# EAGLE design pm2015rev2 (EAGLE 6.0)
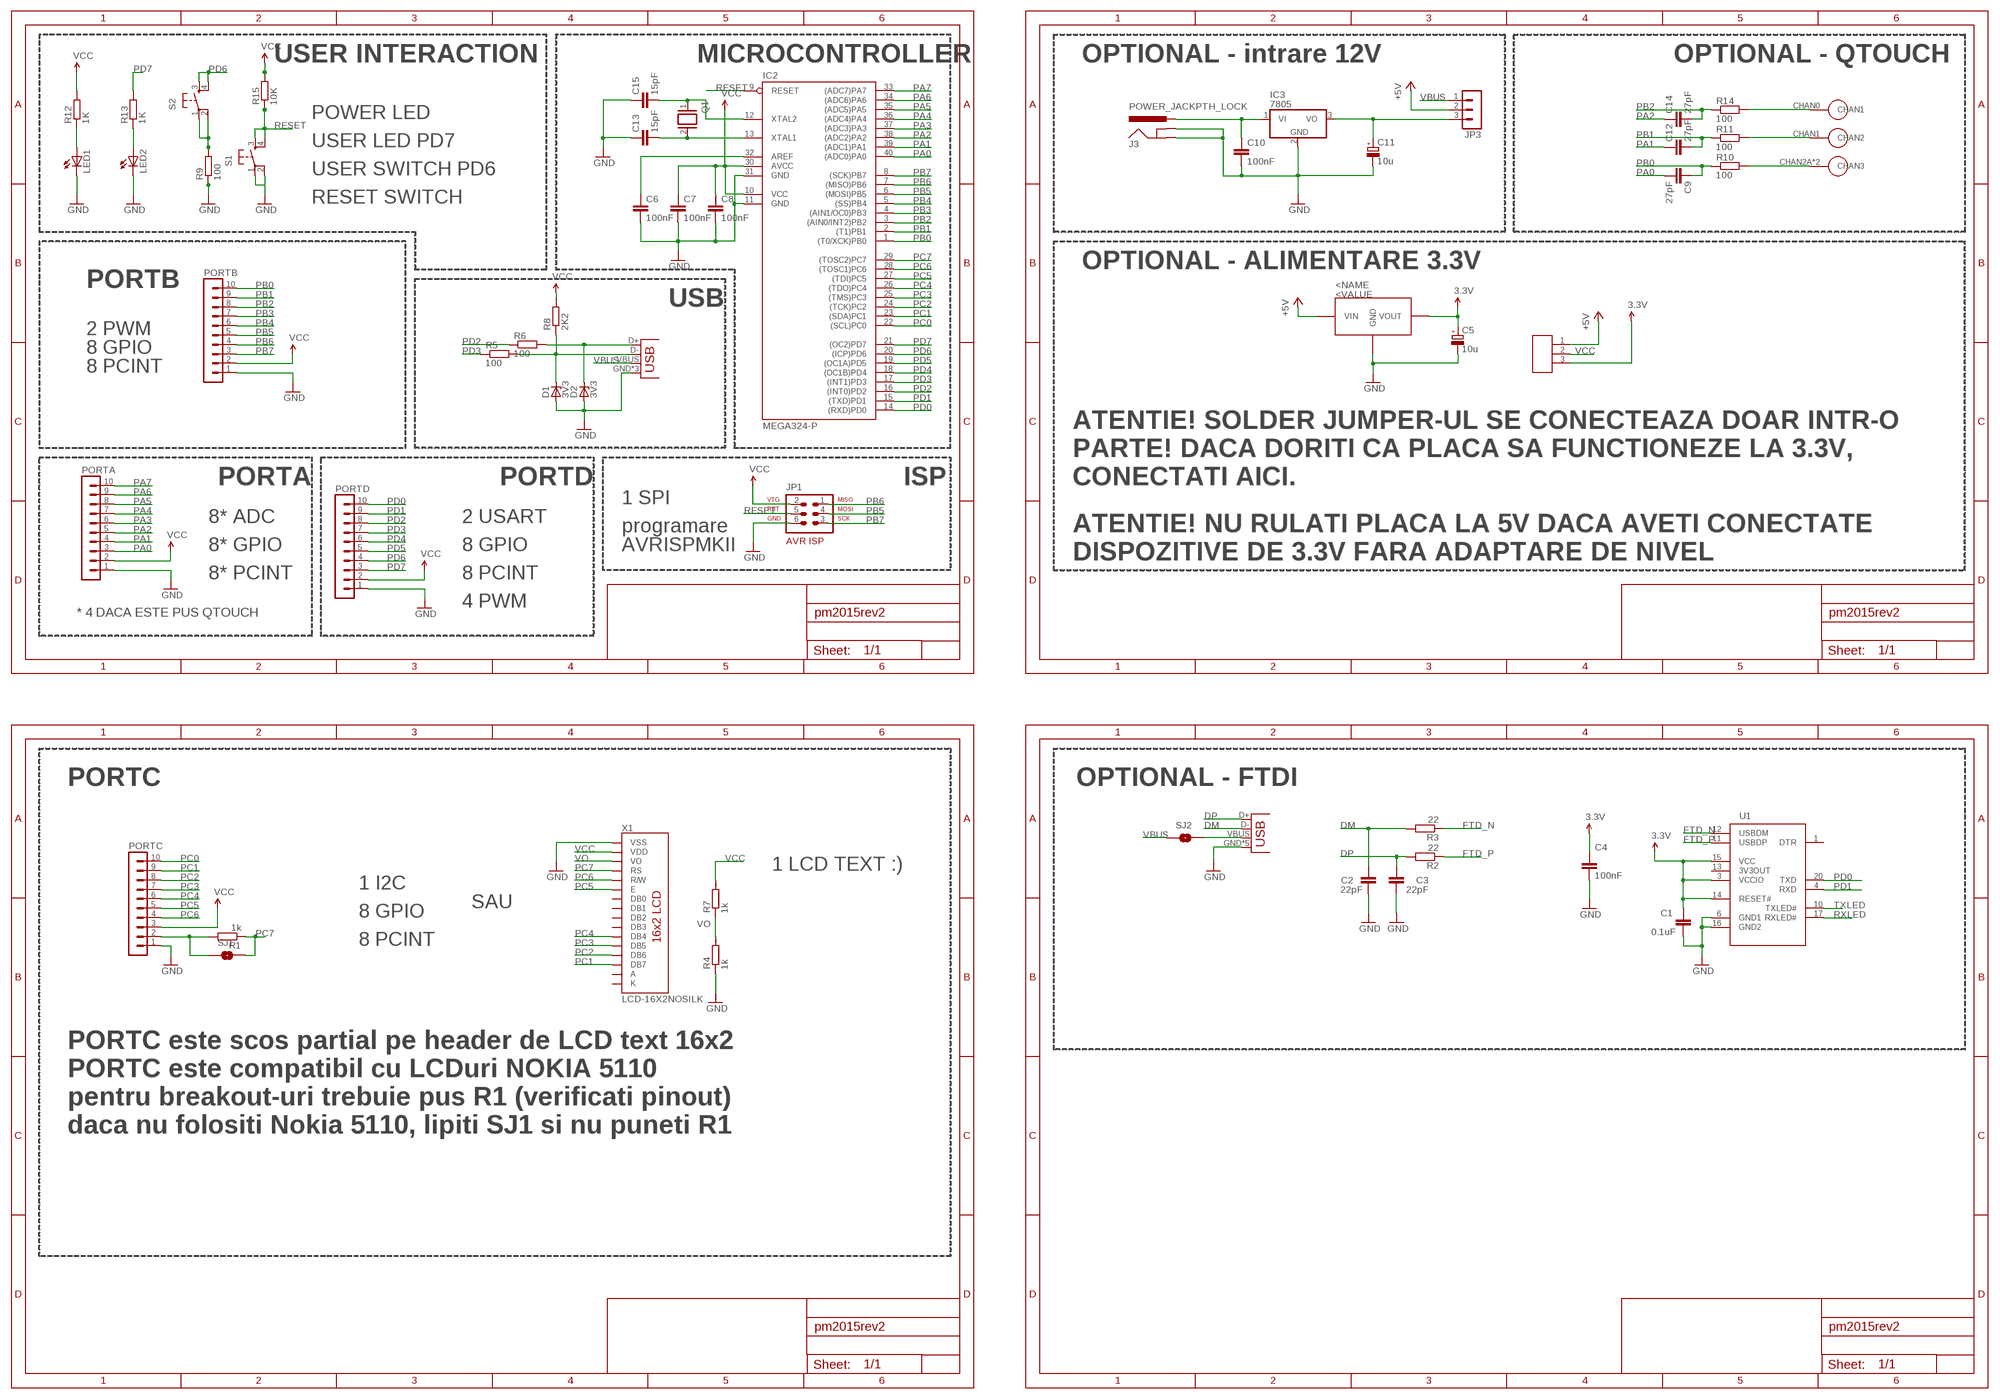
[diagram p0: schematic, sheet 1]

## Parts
C1  0.1uF  C-EUC0603  [C0603]
C2  22pF  C-EUC0603  [C0603]
C3  22pF  C-EUC0603  [C0603]
C4  100nF  C-EUC0603  [C0603]
C5  10u  CPOL-EUE2.5-5  [E2,5-5]
C6  100nF  C-EUC_PM  [C025-025X050]
C7  100nF  C-EUC_PM  [C025-025X050]
C8  100nF  C-EUC_PM  [C025-025X050]
C9  27pF  C-EUC1206  [C1206]
C10  100nF  C-EU025-025X050  [C025-025X050@1]
C11  10u  CPOL-EUE2.5-5  [E2,5-5]
C12  27pF  C-EUC1206  [C1206]
C13  15pF  C-EUC_PM  [C025-025X050]
C14  27pF  C-EUC1206  [C1206]
C15  15pF  C-EUC_PM  [C025-025X050]
D1  3V3  ZENER-DIODEDO34-7  [DO34Z7]
D2  3V3  ZENER-DIODEDO34-7  [DO34Z7]
IC1  LE33  [TO92]
IC2  MEGA324-P  MEGA16-P  [DIL40]
IC3  7805  7805TNH  [TO22H_NOHOLE]
J1  USBMICROUSB  [ZX62D-B-5PA8]
J2  USBPTH  [USB-B-PTH]
J3  POWER_JACKPTH_LOCK  [POWER_JACK_PTH_LOCK]
JP1  AVR-ISP-6  [AVR-ISP-6]
JP2  SJUMPER  [SJUMPER_PACK]
JP3  MA03-1  [MA03-1]
LED1  TLLR4400  [LED3MM]
LED2  TLLR4400  [LED3MM]
PORTA  MA10-1  [MA10-1]
PORTB  MA10-1  [MA10-1]
PORTC  MA10-1  [MA10-1]
PORTD  MA10-1  [MA10-1]
Q1  XTAL/S  [QS]
R1  1k  R-EU_0204/7  [0204/7]
R2  22  R-EU_R0603  [R0603]
R3  22  R-EU_R0603  [R0603]
R4  1k  R-EU_0204/7  [0204/7]
R5  100  R-EU_0204/7  [0204/7]
R6  100  R-EU_0204/7  [0204/7]
R7  1k  R-EU_0204/7  [0204/7]
R8  2K2  R-EU_0204/7  [0204/7]
R9  100  R-EU_0204/7  [0204/7]
R10  100  R-EU_M1206  [M1206]
R11  100  R-EU_M1206  [M1206]
R12  1K  R-EU_0204/7  [0204/7]
R13  1K  R-EU_0204/7  [0204/7]
R14  100  R-EU_M1206  [M1206]
R15  10K  R-EU_0204/7  [0204/7]
S1  TAC_SWITCHPTH  [TACTILE-PTH]
S2  TAC_SWITCHPTH  [TACTILE-PTH]
SJ1  SOLDERJUMPERNC  [SJ-NC]
SJ2  SOLDERJUMPERNC  [SJ-NC]
U1  FT231XS  [SSOP20]
U$1  QT_SLIDER  [QT_SLIDER]
X1  LCD-16X2NOSILK  [LCD-16X2_NOSILK]

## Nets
3.3V: C1.1 C4.1 C5.+ IC1.3(VOUT) JP2.3 U1.3(VCCIO) U1.14(RESET#) U1.15(VCC)
+5V: IC1.1(VIN) JP2.1 JP3.2
DM: C2.2 J1.D- R3.2
DP: C3.2 J1.D+ R2.2
FTD_N: R3.1 U1.12(USBDM)
FTD_P: R2.1 U1.11(USBDP)
GND: C1.2 C2.1 C3.1 C4.2 C5.- C6.2 C7.2 C8.2 C10.2 C11.- C13.1 C15.1 D1.A D2.A IC1.2(GND) IC2.11(GND) IC2.31(GND) IC3.2(GND) J1.GND J1.P$8(GND) J1.P$9(GND) J1.P$10(GND) J1.P$11(GND) J2.GND J2.P$1(GND) J2.P$2(GND) J3.GND J3.GNDBREAK JP1.6 LED1.K(C) LED2.K(C) PORTA.1 PORTB.1 PORTC.1 PORTD.1 R4.1 R9.1 S1.1 S1.2 U1.6(GND1) U1.16(GND2) X1.1(VSS)
N$1: LED2.A R13.1
N$2: LED1.A R12.1
N$3: PORTC.2 R1.2 SJ1.1
N$4: J1.VBUS SJ2.2
N$5: R14.2 U$1.CHAN0(CHAN1)
N$6: R11.2 U$1.CHAN1(CHAN2)
N$7: R10.2 U$1.CHAN2A(CHAN3) U$1.CHAN2B(CHAN3)
N$14: D2.C J2.D+ R6.2
N$15: D1.C J2.D- R5.2 R8.1
N$16: C10.1 IC3.1(VI) J3.PWR
N$17: R9.2 S2.1 S2.2
N$18: C11.+ IC3.3(VO) JP3.3
N$20: C6.1 IC2.32(AREF)
N$21: C13.2 IC2.13(XTAL1) Q1.2
N$22: C15.2 IC2.12(XTAL2) Q1.1
PA0: C9.2 IC2.40((ADC0)PA0) PORTA.3
PA1: C12.1 IC2.39((ADC1)PA1) PORTA.4
PA2: C14.1 IC2.38((ADC2)PA2) PORTA.5
PA3: IC2.37((ADC3)PA3) PORTA.6
PA4: IC2.36((ADC4)PA4) PORTA.7
PA5: IC2.35((ADC5)PA5) PORTA.8
PA6: IC2.34((ADC6)PA6) PORTA.9
PA7: IC2.33((ADC7)PA7) PORTA.10
PB0: C9.1 IC2.1((T0/XCK)PB0) PORTB.10 R10.1
PB1: C12.2 IC2.2((T1)PB1) PORTB.9 R11.1
PB2: C14.2 IC2.3((AIN0/INT2)PB2) PORTB.8 R14.1
PB3: IC2.4((AIN1/OC0)PB3) PORTB.7
PB4: IC2.5((SS)PB4) PORTB.6
PB5: IC2.6((MOSI)PB5) JP1.4 PORTB.5
PB6: IC2.7((MISO)PB6) JP1.1 PORTB.4
PB7: IC2.8((SCK)PB7) JP1.3 PORTB.3
PC0: IC2.22((SCL)PC0) PORTC.10
PC1: IC2.23((SDA)PC1) PORTC.9 X1.14(DB7)
PC2: IC2.24((TCK)PC2) PORTC.8 X1.13(DB6)
PC3: IC2.25((TMS)PC3) PORTC.7 X1.12(DB5)
PC4: IC2.26((TDO)PC4) PORTC.6 X1.11(DB4)
PC5: IC2.27((TDI)PC5) PORTC.5 X1.6(E)
PC6: IC2.28((TOSC1)PC6) PORTC.4 X1.5(R/W)
PC7: IC2.29((TOSC2)PC7) R1.1 SJ1.2 X1.4(RS)
PD0: IC2.14((RXD)PD0) PORTD.10 U1.20(TXD)
PD1: IC2.15((TXD)PD1) PORTD.9 U1.4(RXD)
PD2: IC2.16((INT0)PD2) PORTD.8 R6.1
PD3: IC2.17((INT1)PD3) PORTD.7 R5.1
PD4: IC2.18((OC1B)PD4) PORTD.6
PD5: IC2.19((OC1A)PD5) PORTD.5
PD6: IC2.20((ICP)PD6) PORTD.4 S2.3 S2.4
PD7: IC2.21((OC2)PD7) PORTD.3 R13.2
RESET: IC2.9(RESET) JP1.5 R15.1 S1.3 S1.4
RXLED: U1.17(RXLED#)
TXLED: U1.10(TXLED#)
VBUS: J2.VBUS JP3.1 SJ2.1
VCC: C7.1 C8.1 IC2.10(VCC) IC2.30(AVCC) JP1.2 JP2.2 PORTA.2 PORTB.2 PORTC.3 PORTD.2 R7.2 R8.2 R12.2 R15.2 X1.2(VDD)
VO: R4.2 R7.1 X1.3(VO)
Unconnected: U1.1(DTR) U1.13(3V3OUT) X1.7(DB0) X1.8(DB1) X1.9(DB2) X1.10(DB3)

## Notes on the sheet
- USER INTERACTION | MICROCONTROLLER | OPTIONAL - intrare 12V | OPTIONAL - QTOUCH
- POWER LED
- USER LED PD7
- USER SWITCH PD6
- RESET SWITCH
- OPTIONAL - ALIMENTARE 3.3V
- PORTB
- USB
- 2 PWM
- 8 GPIO
- 8 PCINT
- ATENTIE! SOLDER JUMPER-UL SE CONECTEAZA DOAR INTR-O
- PARTE! DACA DORITI CA PLACA SA FUNCTIONEZE LA 3.3V,
- PORTA | PORTD | ISP | CONECTATI AICI.
- 1 SPI
- 8* ADC | 2 USART
- programare | ATENTIE! NU RULATI PLACA LA 5V DACA AVETI CONECTATE
- 8* GPIO | 8 GPIO | AVRISPMKII
- DISPOZITIVE DE 3.3V FARA ADAPTARE DE NIVEL
- 8* PCINT | 8 PCINT
- 4 PWM
- * 4 DACA ESTE PUS QTOUCH
- PORTC | OPTIONAL - FTDI
- 1 LCD TEXT :)
- 1 I2C
- SAU
- 8 GPIO
- 8 PCINT
- PORTC este scos partial pe header de LCD text 16x2
- PORTC este compatibil cu LCDuri NOKIA 5110
- pentru breakout-uri trebuie pus R1 (verificati pinout)
- daca nu folositi Nokia 5110, lipiti SJ1 si nu puneti R1

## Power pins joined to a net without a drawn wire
A: X1.15(A)
K: X1.16(K)

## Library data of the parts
C1-C4 C9 C10 C12 C14 = resistor:C-EU: CAPACITOR, European symbol
C5 C11 = resistor:CPOL-EU: POLARIZED CAPACITOR, European symbol
C6-C8 C13 C15 = 0andrei_custom:C-EU: CAPACITOR, European symbol
D1 D2 = diode:ZENER-DIODE: Z-Diode
IC1 = 0andrei_custom:LE33
IC2 = atmel:MEGA16-P: MICROCONTROLLER 16 Kbytes FLASH 1 kbytes SRAM 512 bytes EEPROM USART 8-channel 10 bit ADC Source: avr.lbr; MPN: ATMEGA16-16PU; OC_FARNELL: 9171142; OC_NEWARK: 01M6885
IC3 = 0andrei_custom:78*: Positive VOLTAGE REGULATOR Source: http://cache.national.com/ds/LM/LM78L05.pdf http://www.fairchildsemi.com/ds/LM/LM7805.pdf
J1 J2 = 0andrei_custom:USB: USB Connectors USB-B-PTH is fully proven SKU : PRT-00139 USB-miniB is fully proven SKU : PRT-00587 USB-A-PCB is untested. USB-A-H is throughly reviewed, but untested. Spark Fun Electronics SKU : PRT-00437 USB-B-SMT is throughly reviewed, but untested. Needs silkscreen touching up. USB-A-S has not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
J3 = SparkFun-Connectors:POWER_JACK: Power Jack This is the standard 5.5mm barrel jack for power. The PTH is the most common, proven, reliable, footprint. The Slot footprint only works if the mill layer is transmitted to the PCB fab house so be warned. Spark Fun Electronics SKU : PRT-00119 SMT: CONN-08106 Mating wall wart : TOL-00298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
JP1 = 0andrei_custom:AVR-ISP-6: AVR ISP-6 Serial Programming Header
JP2 = 0andrei_custom:SJUMPER
JP3 = con-lstb:MA03-1: PIN HEADER; OC_FARNELL: unknown; OC_NEWARK: unknown
LED1 LED2 = led:TLLR4400: Low Current (2mA) LED 3 mm Tinted Diffused Package color RED; MF: VISHAY SEMICONDUCTOR; OC_FARNELL: 1612437
PORTA PORTB PORTC PORTD = con-lstb:MA10-1: PIN HEADER; OC_FARNELL: unknown; OC_NEWARK: unknown
Q1 = special:XTAL/S: CRYSTAL
R1 R4-R9 R12 R13 R15 = 0andrei_custom:R-EU_: RESISTOR, European symbol
R2 R3 R10 R11 R14 = resistor:R-EU_: RESISTOR, European symbol
S1 S2 = SparkFun:TAC_SWITCH: Momentary Switch Button commonly used for reset or general input. Spark Fun Electronics SKU : COM-00097
SJ1 SJ2 = SparkFun-3-2-07:SOLDERJUMPER: Solder Jumper
U1 = 0andrei_custom:FT231XS
U$1 = 0andrei_custom:QT_SLIDER
X1 = 0andrei_custom:LCD-16X2: Standard text-only 16x2 parallel input LCD

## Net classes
1 power: width 0.61 mm

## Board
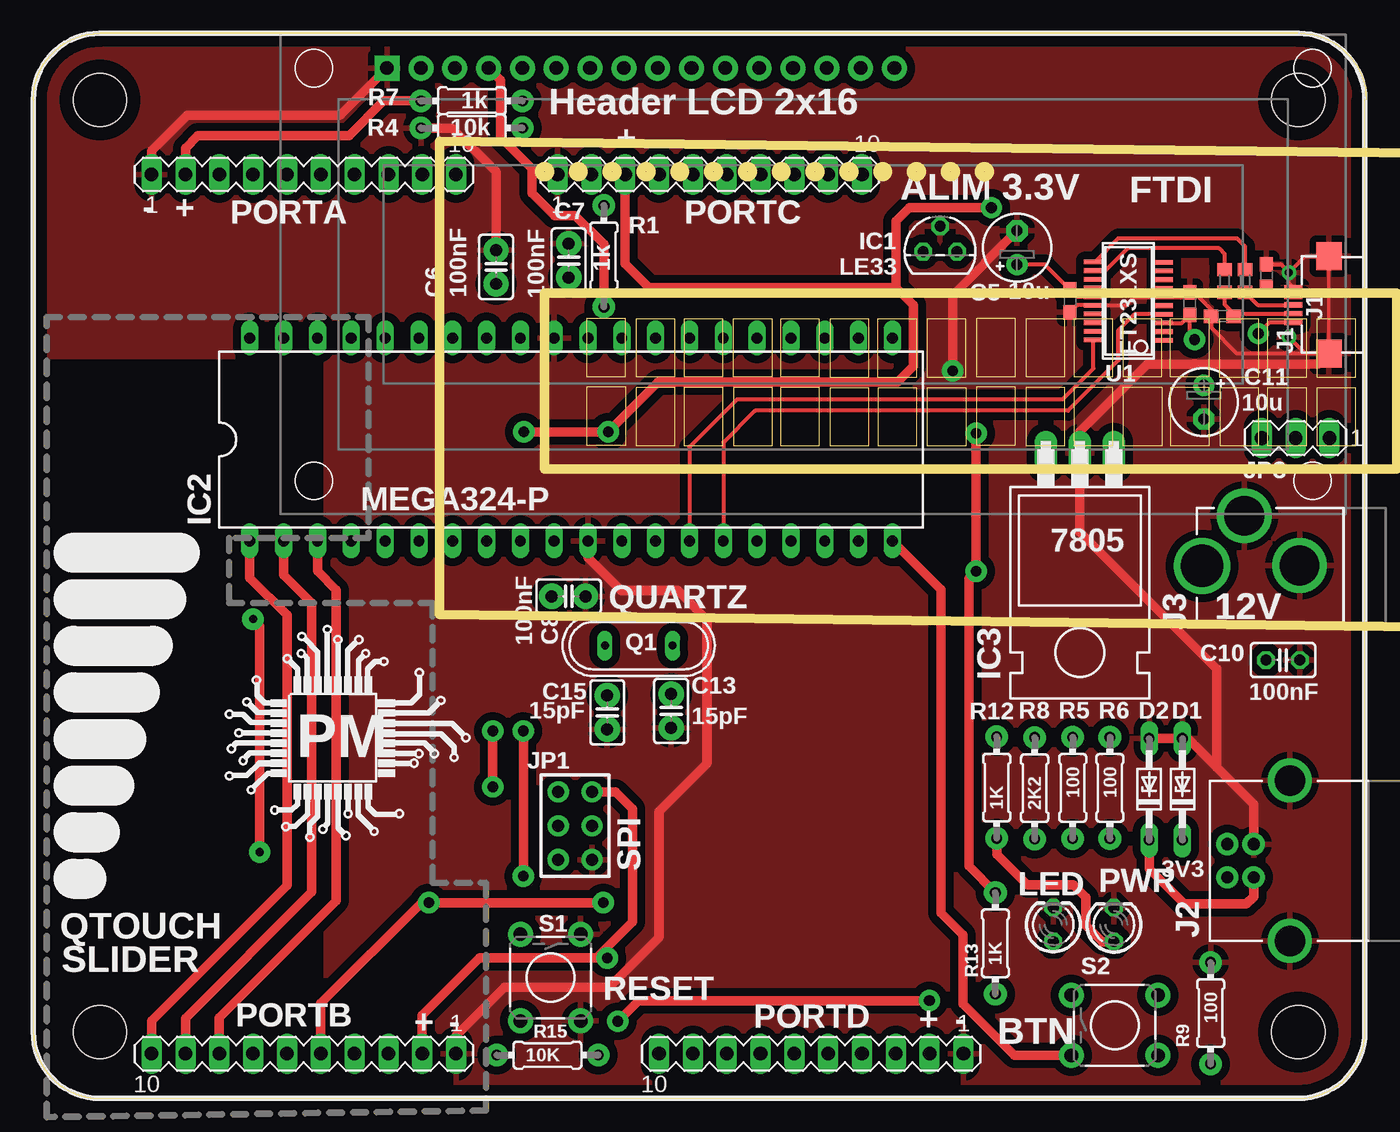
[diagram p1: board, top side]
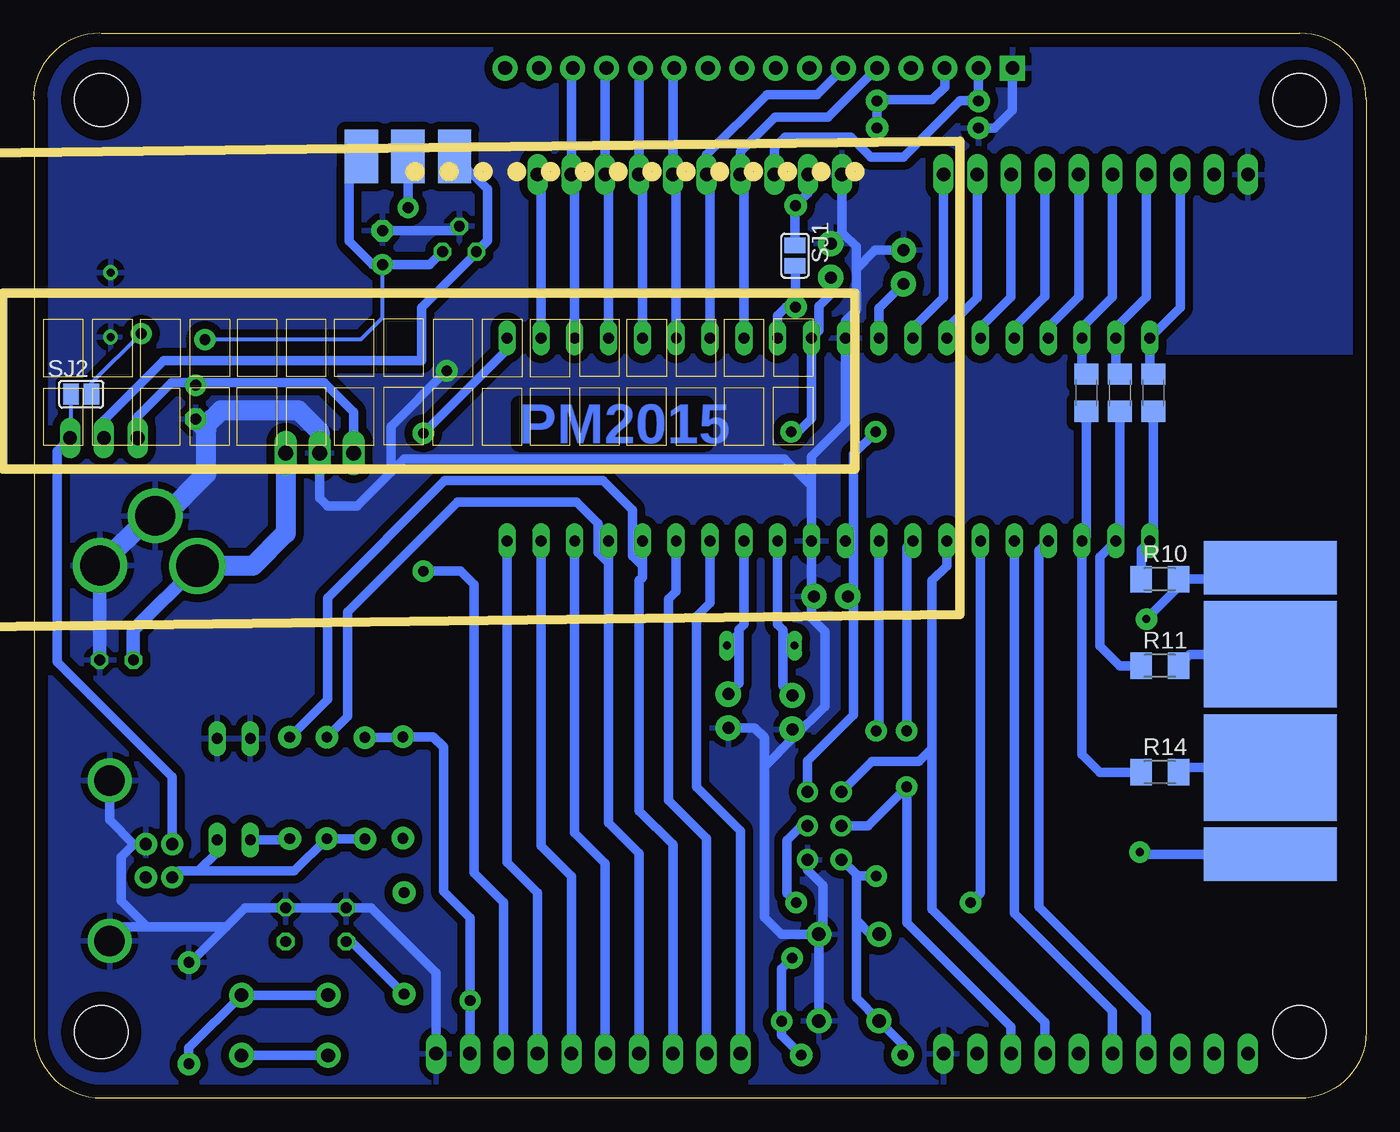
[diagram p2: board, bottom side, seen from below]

Size 100.1 x 80 mm. Coordinates in mm from the lower left corner, seen from the top.
Outline: 100,75 100,5 arc-90 95,0 5,0 arc-90 0,5 0,75 arc-90 5,80 95,80
Outline: 95.1,80 arc-90 100.1,75
Copper layers (1*16): Top 0.035mm / dielectric 1.5mm / Bottom 0.035mm
Design rules: minimum track width 10mil, minimum drill 0.6mm, track to track 0.25mm, track to pad 10mil, pad to pad 0.2mm, via to via 10mil, smd to smd 0mil, copper to edge 40mil, drill to drill 10mil, minimum pad ring 10mil, minimum via ring 8mil, stop-mask expansion 0mil, vias tented up to drill 0mil, thermal gap 20mil
Holes 4 mm at 95,75 5,5 5,75 95,5
Milling: area 38,69.3 to 38.8,70; area 40.6,69.3 to 41.3,70; area 43.1,69.3 to 43.8,70; area 45.7,69.3 to 46.4,70; area 48.2,69.3 to 48.9,70; area 50.7,69.3 to 51.5,70; area 53.3,69.3 to 54,70; area 55.8,69.3 to 56.5,70; area 58.4,69.3 to 59.1,70; area 60.9,69.3 to 61.6,70; area 63.4,69.3 to 64.2,70; area 66,69.3 to 66.7,70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; 8 lines

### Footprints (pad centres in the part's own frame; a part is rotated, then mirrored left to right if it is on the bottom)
C0603 = smd 1.1 x 1: 1 -0.85,0; 2 0.85,0
E2,5-5 = drill 0.813 pad 1.6: + -1.27,0 | drill 0.813 pad 1.6 octagon: - 1.27,0
C025-025X050 = drill 0.9 pad 1.9: 1 -1.27,0; 2 1.27,0
C1206 = smd 1.6 x 1.8: 1 -1.4,0; 2 1.4,0
C025-025X050@1 = drill 0.813 octagon: 1 -1.27,0; 2 1.27,0
DO34Z7 = drill 0.813 long: A 3.81,0; C -3.81,0
TO92 = drill 0.813 octagon: 1 -1.27,0; 2 0,1.905; 3 1.27,0
DIL40 = drill 0.813 long: 1 -24.13,-7.62; 2 -21.59,-7.62; 3 -19.05,-7.62; 4 -16.51,-7.62; 5 -13.97,-7.62; 6 -11.43,-7.62; 7 -8.89,-7.62; 8 -6.35,-7.62; 9 -3.81,-7.62; 10 -1.27,-7.62; 11 1.27,-7.62; 12 3.81,-7.62; 13 6.35,-7.62; 14 8.89,-7.62; 15 11.43,-7.62; 16 13.97,-7.62; 17 16.51,-7.62; 18 19.05,-7.62; 19 21.59,-7.62; 20 24.13,-7.62; 21 24.13,7.62; 22 21.59,7.62; 23 19.05,7.62; 24 16.51,7.62; 25 13.97,7.62; 26 11.43,7.62; 27 8.89,7.62; 28 6.35,7.62; 29 3.81,7.62; 30 1.27,7.62; 31 -1.27,7.62; 32 -3.81,7.62; 33 -6.35,7.62; 34 -8.89,7.62; 35 -11.43,7.62; 36 -13.97,7.62; 37 -16.51,7.62; 38 -19.05,7.62; 39 -21.59,7.62; 40 -24.13,7.62
TO22H_NOHOLE = drill 1.118 long: 1 -2.54,-10.16; 2 0,-10.16; 3 2.54,-10.16
ZX62D-B-5PA8 = smd 0.4 x 1.35: D+ 0,2.675; D- -0.65,2.675; GND 1.3,2.675; ID 0.65,2.675; VBUS -1.3,2.675 | drill 0.6: P$8 -2.425,3; P$9 2.425,3 | smd 2.1 x 1.9: P$10 -3.65,0; P$11 3.65,0
USB-B-PTH = drill 0.914 pad 1.676: D+ 0,1.25; D- 1.981,1.25; GND 0,-1.25; VBUS 1.981,-1.25 | drill 2.286: P$1 -2.718,-6.02; P$2 -2.718,6.02
POWER_JACK_PTH_LOCK = drill 2.997 pad 4.115: GND 0.025,6.557; GNDBREAK 3.762,10.7 | drill 3.2 pad 4.115: PWR 0,13.878
AVR-ISP-6 = drill 0.9 pad 1.6: 1 -2.54,-1.27; 2 -2.54,1.27; 3 0,-1.27; 4 0,1.27; 5 2.54,-1.27; 6 2.54,1.27
SJUMPER_PACK = smd 2.5 x 4: 1 -3.54,0; 2 -0.04,0; 3 3.46,0
MA03-1 = drill 1.016 long: 1 -2.54,0; 2 0,0; 3 2.54,0
LED3MM = drill 0.813 octagon: A -1.27,0; K 1.27,0
MA10-1 = drill 1.016 long: 1 -11.43,0; 2 -8.89,0; 3 -6.35,0; 4 -3.81,0; 5 -1.27,0; 6 1.27,0; 7 3.81,0; 8 6.35,0; 9 8.89,0; 10 11.43,0
QS = drill 0.61 long: 1 -2.54,0; 2 2.54,0
0204/7 = drill 0.813 pad 1.7: 1 -3.81,0; 2 3.81,0
R0603 = smd 1 x 1.1: 1 -0.85,0; 2 0.85,0
M1206 = smd 1.6 x 2: 1 -1.4,0; 2 1.4,0
TACTILE-PTH = drill 1.016 pad 1.88: 1 -3.251,2.261; 2 3.251,2.261; 3 -3.251,-2.261; 4 3.251,-2.261
SJ-NC = smd 1.168 x 1.6: 1 -0.762,0; 2 0.762,0
SSOP20 = smd 0.348 x 1.397: 1 -2.955,-2.64; 2 -2.305,-2.64; 3 -1.655,-2.64; 4 -1.005,-2.64; 5 -0.355,-2.64; 6 0.295,-2.64; 7 0.945,-2.64; 8 1.595,-2.64; 9 2.245,-2.64; 10 2.895,-2.64; 11 2.925,2.64; 12 2.275,2.64; 13 1.625,2.64; 14 0.975,2.64; 15 0.325,2.64; 16 -0.325,2.64; 17 -0.975,2.64; 18 -1.625,2.64; 19 -2.275,2.64; 20 -2.925,2.64
QT_SLIDER = smd 8 x 10: CHAN0 -4.25,0; CHAN1 4.25,0 | smd 4 x 10: CHAN2A 10.75,0; CHAN2B -10.75,0
LCD-16X2_NOSILK = drill 1.016 pad 1.88 square: 1 -32,15.5 | drill 1.016 pad 1.88: 2 -29.46,15.5; 3 -26.92,15.5; 4 -24.38,15.5; 5 -21.84,15.5; 6 -19.3,15.5; 7 -16.76,15.5; 8 -14.22,15.5; 9 -11.68,15.5; 10 -9.14,15.5; 11 -6.6,15.5; 12 -4.06,15.5; 13 -1.52,15.5; 14 1.02,15.5; 15 3.56,15.5; 16 6.1,15.5

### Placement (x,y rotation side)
C1  77.85,59.9 270 top
C2  89.3,58.75 0 top
C3  92.6,61.8 270 top
C4  86.85,59.7 90 top
C5  73.88,63.9 90 top
C6  34.75,62.45 90 top
C7  40.21,62.93 90 top
C8  40.21,37.71 0 top
C9  16,53 90 bottom
C10  93.85,32.93 0 top
C11  87.9,52.3 270 top
C12  18.5,53 270 bottom
C13  47.9,29.1 90 top
C14  21,53 270 bottom
C15  43.1,29 90 top
D1  86.3,23.23 90 top
D2  83.8,23.23 90 top
IC1  68.1,63.6 0 top
IC2  40.39,49.5 0 top
IC3  78.6,38.31 180 top
J1  97.3,59.6 90 top
J2  91.65,17.85 180 top
J3  101.65,40 90 top
JP1  40.69,20.48 270 top
JP2  72,70.75 180 bottom
JP3  94.8,49.6 180 top
LED1  81.15,13.05 90 top
LED2  76.6,13.05 90 top
PORTA  20.32,69.4 0 top
PORTB  20.32,3.36 180 top
PORTC  50.8,69.4 0 top
PORTD  58.42,3.36 180 top
Q1  45.47,34.01 0 top
R1  42.85,63.25 90 top
R2  91,61.4 270 top
R3  89.45,61.4 270 top
R4  32.92,72.89 0 top
R5  78.06,23.32 270 top
R6  80.85,23.32 270 top
R7  32.92,74.92 180 top
R8  75.2,23.3 90 top
R9  88.42,6.41 270 top
R10  15.5,39 0 bottom
R11  15.5,32.5 0 bottom
R12  72.35,23.35 90 top
R13  72.25,11.65 90 top
R14  15.5,24.5 0 bottom
R15  38.62,3.26 0 top
S1  38.85,9.08 270 top
S2  81.21,5.49 0 top
SJ1  42.9,63.3 270 bottom
SJ2  96.5,52.9 0 bottom
U1  82.25,59.9 90 top
U$1  7.2,29.1 90 bottom
X1  58.57,61.89 0 top

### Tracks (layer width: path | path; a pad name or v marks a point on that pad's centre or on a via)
3.3V  (via drill 0.8 pad 1.6)
  Top 0.254: C1.1 78.38,60.22
  Top 0.3: U1.14 U1.15 78.38,60.22 | U1.3 86.25,58.25 C4.1 86.85,57.35 v87.2,57 | C1.1 75.97,62.63 C5.+
  Bottom 0.3: v87.2,57 75.51,57 73.88,58.63 C5.+
  Bottom 0.7: IC1.3 70.34,62.63 C5.+ 74.63,62.63 76.4,64.4 76.4,69.81 JP2.3
+5V
  Bottom 0.7: JP3.2 94.8,50.9 90.3,55.4 70.93,55.4 70.93,59.4 66.83,63.5 IC1.1 66,64.43 66,68.29 JP2.1
DM
  Top 0.3: R3.2 89.45,59.65 90.15,58.95 90.35,58.95 | 90.35,58.95 J1.D- | C2.2 90.35,58.95
DP
  Top 0.3: J1.D+ 91.95,59.6 R2.2 92.2,60.55 C3.2
FTD_N
  Top 0.3: U1.12 80.53,62.17 82.2,63.85 89.05,63.85 89.45,63.45 R3.1
FTD_P
  Top 0.3: U1.11 79.72,62.83 81.5,64.6 90.4,64.6 91,64 R2.1
GND  (via drill 0.8 pad 1.6)
  Top 0.254: J1.P$10 J1.P$11
  Top 0.3: 96.53,63.25 J1.P$11 95.53,63.25 J1.P$9 | J1.P$10 95.53,55.95 | 95.53,55.95 90.4,55.95 88.45,57.9 C2.1 88.45,59.25 87.15,60.55 C4.2 86.5,60.19 U1.6 82.69,60.19 82.08,59.58 U1.16 78.38,59.58 C1.2 | C3.1 93.67,62.65 J1.P$9 | J1.GND 94.3,61.22 J1.P$9 | J1.P$8 95.53,55.95
  Top 0.7: J2.GND 91.65,22.1 88.88,24.88 | D2.A D1.A 86.71,27.04 88.88,24.88 | PORTB.1 31.75,4.7 35.4,8.35 43.25,8.35 47,12.1 47,21.55 50.6,25.15 50.6,35.95 48.4,38.15 44.15,38.15 41.66,40.64 IC2.11 | 88.88,24.88 88.88,32.27 78.6,42.55 IC3.2 78.6,50.1 83.65,55.15 96.5,55.15 J1.P$10 | R4.1 31.46,72.89 34.75,69.6 C6.2 | PORTA.1 8.89,71.19 11.55,73.85 23.03,73.85 X1.1 | v69.05,54.65 69.05,60.34 C5.-
  Bottom 0.7: IC2.11 41.66,46 | 41.66,46 41.66,48.23 39.12,50.77 IC2.31 39.12,58.38 38.3,59.2 38.3,62.3 | 41.66,37.89 41.66,36.09 40.64,35.08 40.64,29.46 43,27.1 | 41.66,37.89 IC2.11 | S1.2 S1.1 | 41.66,44.47 IC2.11 | 41.66,46 43.69,48.03 72.24,48.03 73.24,47.04 | 43,27.1 43.1,27.2 C15.1 | 43,27.1 45.2,24.9 | C8.2 41.66,37.89 | C13.1 45.93,27.83 45.2,27.1 45.2,24.9 | JP1.6 41.96,17.16 40.8,16 40.8,12.64 S1.1 | 85.6,12.9 84.18,14.32 LED1.K LED2.K 74.72,14.32 69.85,9.45 PORTD.1 | 85.6,12.9 91.55,12.9 | 91.55,12.9 93.5,14.85 93.5,18.15 92.55,19.1 | 92.55,19.1 J2.GND | C7.2 39.37,65.04 | 39.37,65.04 PORTC.1 | X1.1 26.57,74.23 27.91,72.89 R4.1 | 38.3,62.3 36.88,63.72 C6.2 | 45.2,24.9 45.2,13.6 43.93,12.33 S1.1 | v69.05,54.65 73.24,50.46 73.24,47.04 | 38.3,62.3 38.3,63.97 39.37,65.04 | 73.24,47.04 75.77,44.5 78,44.5 78.6,45.1 IC3.2 | 91.55,12.9 93.3,12.9 J2.P$2 | J2.P$1 94.37,20.92 92.55,19.1 | IC1.2 68.44,65.17 C5.- | R9.1 88.28,10.22 85.6,12.9
  Bottom 1: C10.2 95.12,40 J3.GND
  Bottom 1.5: 87.1,50.23 87.1,46.9 90.24,43.76 J3.GNDBREAK 91.36,43.76 J3.GND | 87.1,50.23 87.1,50.6 86,51.7 80.2,51.7 78.6,50.1 IC3.2 | C11.- 87.1,50.23
  pour Bottom (isolate 0.6): -2.15,79.63 100.94,79.63 100.94,-2.75 21.68,-2.75 21.68,44.84 21.68,56.05 7.04,56.05 -2.1,56.05 -2.1,79.6
  pour Top (isolate 0.6): -1.8,80.8 101.3,80.8 101.3,0.1 22,0.1 22,55.7 -1.8,55.7
N$1
  Bottom 0.7: LED2.A 76.19,11.78 R13.1
N$2
  Top 0.7: R12.1 72.35,18.35 74.65,16.05 78.1,16.05 79.05,15.1 79.05,13 80.27,11.78 LED1.A
N$3
  Bottom 0.7: PORTC.2 41.91,68 R1.2 42.9,67.01 SJ1.1
N$4  (via drill 0.8 pad 1.6)
  Top 0.3: v92,57.45 92.85,58.3 J1.VBUS
  Bottom 0.3: v92,57.45 95.74,53.71 SJ2.2
N$5
  Bottom 0.7: R14.2 13.75,24.85 U$1.CHAN0
N$6
  Bottom 0.7: R11.2 13.25,33.35 U$1.CHAN1
N$7  (via drill 0.61 pad 1.6)
  Top 0.7: v17,18.5 17,35.5 v16.5,36
  Bottom 0.7: U$1.CHAN2A 8.05,39 R10.2 14.1,38.4 v16.5,36 | U$1.CHAN2B 16.85,18.35 v17,18.5
N$14
  Top 0.7: J2.D+ 91.65,15.15 91.1,14.6 86.45,14.6 83.8,17.25 D2.C
  Bottom 0.7: R6.2 80.95,19.42 D2.C
N$15
  Bottom 0.7: J2.D- 89.19,17.08 87.7,17.08 | 87.7,17.08 80.49,17.08 R5.2 78.03,19.49 R8.1 | D1.C 86.3,18.48 87.7,17.08
N$16
  Bottom 1: C10.1 92.58,35.19 J3.PWR
  Bottom 1.5: J3.PWR 83.6,40 81.14,42.46 IC3.1
N$17
  Bottom 0.7: S2.1 S2.2 88.42,3.8 R9.2
N$18
  Bottom 0.7: 88.1,53.77 78.27,53.77 76.06,51.56 IC3.3 | C11.+ 88.1,53.77 | 88.1,53.77 89.69,53.77 92.26,51.2 JP3.3
N$20
  Bottom 0.7: IC2.32 36.58,59.35 C6.1
N$21
  Bottom 0.7: IC2.13 46.74,35.58 47.1,35.22 47.1,34.92 | 47.1,34.92 47.1,31.17 C13.2 | Q1.2 47.1,34.92
N$22
  Bottom 0.7: IC2.12 44.2,35.58 43.8,35.19 43.8,34.8 | 43.8,34.8 43.8,30.97 C15.2 | Q1.1 43.71,34.8 43.8,34.8
PA0
  Bottom 0.7: PORTA.3 13.97,59.4 IC2.40 16.26,54.66 C9.2
PA1
  Bottom 0.7: PORTA.4 16.51,60.19 18.8,57.9 IC2.39 18.8,54.7 C12.1
PA2
  Bottom 0.7: PORTA.5 19.05,60.2 21.34,57.91 IC2.38 21.34,54.74 C14.1
PA3
  Bottom 0.7: PORTA.6 21.59,60.21 23.88,57.92 IC2.37
PA4
  Bottom 0.7: PORTA.7 24.13,60.22 26.42,57.93 IC2.36
PA5
  Bottom 0.7: PORTA.8 26.67,60.18 28.96,57.89 IC2.35
PA6
  Bottom 0.7: PORTA.9 29.21,60.14 31.5,57.85 IC2.34
PA7
  Bottom 0.7: PORTA.10 31.75,60.15 34.04,57.86 IC2.33
PB0
  Top 0.7: PORTB.10 8.89,5.84 19.05,16 19.05,36.3 16.26,39.09 IC2.1
  Bottom 0.7: R10.1 16.9,41.23 IC2.1 16,42.13 C9.1
PB1
  Top 0.7: PORTB.9 11.43,6.03 20.9,15.5 20.9,37.2 18.8,39.3 IC2.2
  Bottom 0.7: R11.1 18.5,32.5 20,34 20,40.67 IC2.2 18.5,42.17 C12.2
PB2
  Top 0.7: PORTB.8 13.97,6.07 22.75,14.85 22.75,38.2 21.34,39.61 IC2.3
  Bottom 0.7: R14.1 20,24.5 21.34,25.84 IC2.3 21,42.21 C14.2
PB3
  Bottom 0.7: PORTB.7 16.51,6.31 24.6,14.4 24.6,41.15 IC2.4
PB4
  Bottom 0.7: PORTB.6 19.05,6.55 26.42,13.92 IC2.5
PB5  (via drill 0.8 pad 1.6)
  Top 0.7: v42.8,14.7 v29.7,14.7 29.15,14.7 21.59,7.14 PORTB.5
  Bottom 0.7: JP1.4 42.42,20.48 43.5,19.4 43.5,15.4 v42.8,14.7 | IC2.6 28.96,15.44 v29.7,14.7
PB6
  Bottom 0.7: IC2.7 31.5,40 32.6,38.9 32.6,26.3 | 32.6,26.3 33.6,25.3 37.14,25.3 JP1.1 | PORTB.4 24.13,5.73 32.6,14.2 32.6,26.3
PB7  (via drill 0.8 pad 1.6)
  Top 0.7: v34.5,27.6 v34.5,23.4
  Bottom 0.7: IC2.8 34.5,41.41 v34.5,27.6 | JP1.3 37.42,20.48 v34.5,23.4 34.5,13.2 26.67,5.37 PORTB.3
PC0
  Bottom 0.7: IC2.22 61.98,69.15 PORTC.10
PC1
  Bottom 0.7: X1.14 59.69,77.29 PORTC.9 59.44,69.15 IC2.23
PC2
  Bottom 0.7: X1.13 57.15,77.29 PORTC.8 56.9,69.15 IC2.24
PC3
  Bottom 0.7: X1.12 54.61,77.29 PORTC.7 54.36,69.15 IC2.25
PC4
  Bottom 0.7: X1.11 52.07,77.29 PORTC.6 51.82,69.15 IC2.26
PC5
  Bottom 0.7: X1.6 41.26,75.4 45,75.4 49.53,70.87 PORTC.5 49.28,69.15 IC2.27
PC6
  Bottom 0.7: X1.5 40.42,73.7 44.4,73.7 46.99,71.11 PORTC.4 46.74,69.15 IC2.28
PC7
  Top 0.7: R1.1 42.85,64.15 40.7,66.3 39.15,66.3 37.45,68 37.45,69.85 35.1,72.2 35.1,76.48 X1.4
  Bottom 0.7: IC2.29 44.2,58.8 43.56,59.44 R1.1 42.85,62.49 SJ1.2
PD0
  Top 0.3: IC2.14 49.28,48.93 52.85,52.5 77.28,52.5 79.61,54.83 U1.20
  Bottom 0.7: IC2.14 49.28,37.22 50.3,36.2 50.3,23.4 46.99,20.09 PORTD.10
PD1
  Top 0.3: U1.4 82.69,58.89 81.5,57.7 81.5,55.45 77.7,51.65 54.2,51.65 51.82,49.27 IC2.15
  Bottom 0.7: IC2.15 51.82,38.08 52.4,37.5 52.4,22.4 49.53,19.53 PORTD.9
PD2
  Bottom 0.7: IC2.16 54.36,40 | 54.36,40 54.36,39.14 54.6,38.9 54.6,21.6 52.07,19.07 PORTD.8 | 54.36,40 55.1,40.74 55.1,44.2 57.3,46.4 69.19,46.4 78,37.59 78,29.99 R6.1
PD3
  Bottom 0.7: IC2.17 56.9,40.2 | 56.9,40.2 56.9,20.7 54.61,18.41 PORTD.7 | 56.9,40.2 57.7,41 57.7,43.2 59.3,44.8 68.25,44.8 76.5,36.55 76.5,28.69 R5.1
PD4
  Bottom 0.7: IC2.18 59.44,19.94 57.15,17.65 PORTD.6
PD5
  Bottom 0.7: IC2.19 61.98,18.98 59.69,16.69 PORTD.5
PD6
  Top 0.7: S2.3 73.67,3.23 69.8,7.1 69.8,12.3 68.15,13.95 68.15,38.24 IC2.20
  Bottom 0.7: IC2.20 64.52,17.72 62.23,15.43 PORTD.4 | S2.3 S2.4
PD7  (via drill 0.8 pad 1.6)
  Top 0.7: v70.8,49.97 v70.8,39.6 70.25,39.05 70.25,17.46 R13.2
  Bottom 0.7: v70.8,49.97 64.52,56.25 IC2.21 | PORTD.3 64.77,14.72 67,16.95 67,38.6 68,39.6 v70.8,39.6
RESET  (via drill 0.8 pad 1.6)
  Top 0.7: v36.8,27.6 v36.8,16.7
  Bottom 0.7: 38.3,16.82 38.3,13.4 | 38.3,13.4 38.3,7.54 S1.4 34.81,4.05 R15.1 | IC2.9 36.58,27.88 36.8,27.65 v36.8,27.6 | JP1.5 38.3,16.82 | S1.3 37.23,12.33 38.3,13.4 | v36.8,16.7 38.18,16.7 38.3,16.82
VBUS
  Bottom 0.3: JP3.1 97.26,49.68 SJ2.1
  Bottom 0.7: J2.VBUS 89.67,24.17 98.3,32.8 98.3,48.64 JP3.1
VCC  (via drill 0.8 pad 1.6)
  Top 0.7: v36.83,50.06 v43.18,50.06 46.92,53.8 64.9,53.8 66.1,55 66.1,59.6 64.8,60.9 | JP1.2 43.73,23.02 45,21.75 45,13.25 42.3,10.55 | 42.3,10.55 33.5,10.55 29.21,6.26 PORTB.2 | v67.3,7.35 45.45,7.35 v43.9,5.8 | 42.3,10.55 v43.1,10.55 | PORTA.2 11.43,71.38 12.35,72.3 23.7,72.3 26.32,74.92 R7.2 | PORTC.3 44.45,62.7 46.25,60.9 64.8,60.9 | v71.95,66.9 65.8,66.9 64.8,65.9 64.8,60.9
  Bottom 0.7: v36.83,50.06 38.5,48.39 38.5,42.49 | v43.18,50.06 42.67,50.06 41.66,51.08 IC2.30 41.1,57.67 41.1,59.5 40.21,60.39 C7.1 | 38.5,38.15 38.5,28.8 41.96,25.34 JP1.2 | 38.5,38.15 38.5,42.49 | IC2.10 38.5,42.49 | C8.1 38.5,38.15 | R8.2 72.4,27.11 R12.2 70.06,27.16 69.3,26.4 69.3,15.55 67.3,13.55 v67.3,7.35 v67.31,7.34 PORTD.2 | v43.1,10.55 43.9,9.75 v43.9,5.8 43.9,4.73 R15.2 | X1.2 R7.2 30.53,74.92 34.75,70.7 37.2,70.7 38.7,72.2 43.65,72.2 44.45,71.4 PORTC.3 | v71.95,66.9 v71.96,66.91 JP2.2
VO
  Bottom 0.7: R4.2 R7.1 36.66,75 32.6,75 31.65,75.95 X1.3

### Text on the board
Bottom: PM2015
tPlace: Header LCD 2x16 | ALIM 3.3V | FTDI | PORTA | PORTC | QUARTZ | 12V | PM | SPI | PWR | LED | QTOUCH | SLIDER | RESET | PORTB | PORTD | BTN
tNames: - | + | - | + | + | - | + | -
tDocu: Optional | alimentare 3.3V | Optional | alimentare 12V | Optional | QTouch
_tsilk: 1k | R7 | Header LCD 2x16 | R4 | 10k | - | + | ALIM 3.3V | FTDI | - | + | PORTA | C7 | PORTC | R1 | IC1 | 1k | LE33 | C6 | 100nF | 100nF | C5 | 10u | J1 | FT231XS | U1 | C11 | 10u | JP3 | MEGA324-P | IC2 | 7805 | QUARTZ | 12V | J3 | 100nF | C8 | Q1 | C10 | IC3 | C15 | C13 | 100nF | 15pF | R8 | R5 | R6 | D2 | D1 | 15pF | R12 | PM | JP1 | 100 | 100 | 1K | 2K2 | SPI | 3V3 | PWR | LED | QTOUCH | S1 | J2 | 1K | SLIDER | R13 | S2 | 100 | RESET | R9 | PORTB | + | - | R15 | PORTD | + | - | BTN | 10K
_bsilk: SJ1 | SJ2 | R10 | 100 | R11 | 100 | R14 | 100
215bmp: D:/Downloads/logo.bmp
